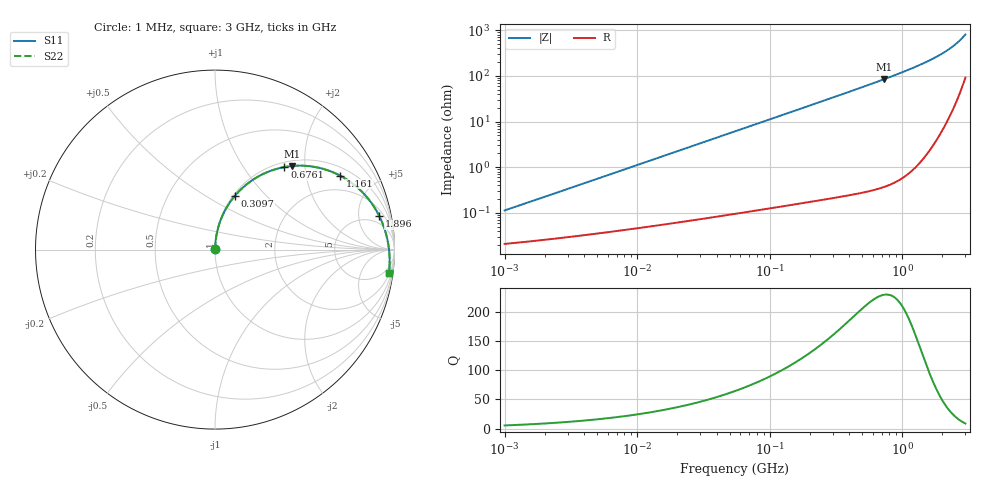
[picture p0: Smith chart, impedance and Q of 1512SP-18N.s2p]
# MHz  S  MA  R  50
!Freq  MagS11  AngS11  MagS21  AngS21  MagS12  AngS12  MagS22  AngS22
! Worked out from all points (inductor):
!   801 points, 1 MHz to 3 GHz, reference 50 ohm
!   read as one part in series: L = 17.7 nH near 1.041 MHz
!   highest Q = 229 at 732.5 MHz (marker M1), where L = 18.4 nH
!   S11 on the Smith chart (normalised r, x): 1 MHz: 1.00, +0.00; 309.7 MHz: 1.02, +0.68; 676.1 MHz: 1.09, +1.56; 1.161 GHz: 1.31, +3.14; 1.896 GHz: 3.05, +8.95; 3 GHz: 2, -15
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1  0.001097 79.0  0.9998 -0.1  0.9998 -0.1  0.001097 79.0
3.824029  0.00413 85.3  0.9997 -0.3  0.9997 -0.3  0.00413 85.3
14.47755  0.01559 87.1  0.9993 -1.0  0.9993 -1.0  0.01559 87.1
30.36588  0.03268 86.7  0.9987 -2.0  0.9987 -2.0  0.03268 86.7
54.81117  0.05891 85.5  0.9973 -3.6  0.9973 -3.6  0.0589 85.5
112.6848  0.1205 82.0  0.9914 -7.4  0.9914 -7.4  0.1204 82.0
209.5995  0.2206 75.9  0.9737 -13.6  0.9737 -13.6  0.2205 75.9
309.692  0.3179 69.8  0.9461 -19.8  0.9461 -19.8  0.3179 69.8
382.1383  0.3835 65.5  0.9214 -24.2  0.9214 -24.2  0.3834 65.5
462.1861  0.4506 61.0  0.8904 -28.7  0.8904 -28.7  0.4504 61.0
559.0017  0.5237 55.8  0.8494 -33.9  0.8494 -33.9  0.5236 55.8
676.0976  0.6008 50.0  0.7968 -39.8  0.7968 -39.8  0.6006 50.0
732.4649  0.6336 47.3  0.7709 -42.4  0.7709 -42.4  0.6334 47.3
793.5315  0.6662 44.6  0.7429 -45.1  0.7429 -45.1  0.666 44.6
959.7552  0.7412 37.8  0.6679 -51.9  0.6679 -51.9  0.7409 37.8
1160.798  0.8094 30.7  0.5829 -59.0  0.5829 -59.0  0.809 30.7
1461.308  0.8783 21.7  0.4709 -67.8  0.4709 -67.8  0.8779 21.7
1895.694  0.9348 11.4  0.3395 -77.5  0.3395 -77.5  0.9344 11.4
2159.143  0.9542 6.2  0.2746 -82.2  0.2746 -82.2  0.9538 6.2
2410.462  0.9661 1.7  0.221 -85.9  0.221 -85.9  0.9658 1.7
2637.697  0.973 -2.0  0.1785 -88.5  0.1785 -88.5  0.9728 -2.0
3000  0.9785 -7.5  0.121 -90.8  0.121 -90.8  0.9785 -7.5
